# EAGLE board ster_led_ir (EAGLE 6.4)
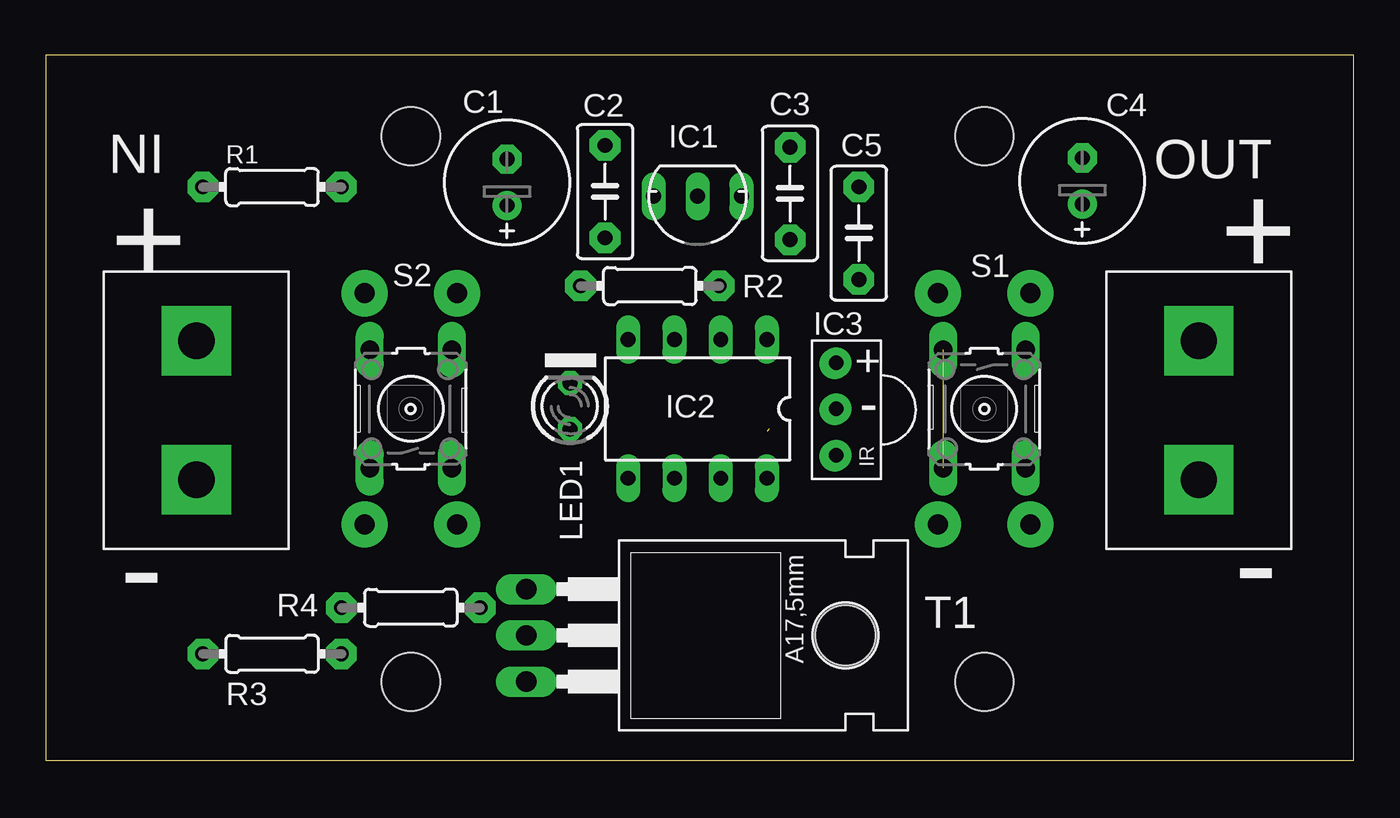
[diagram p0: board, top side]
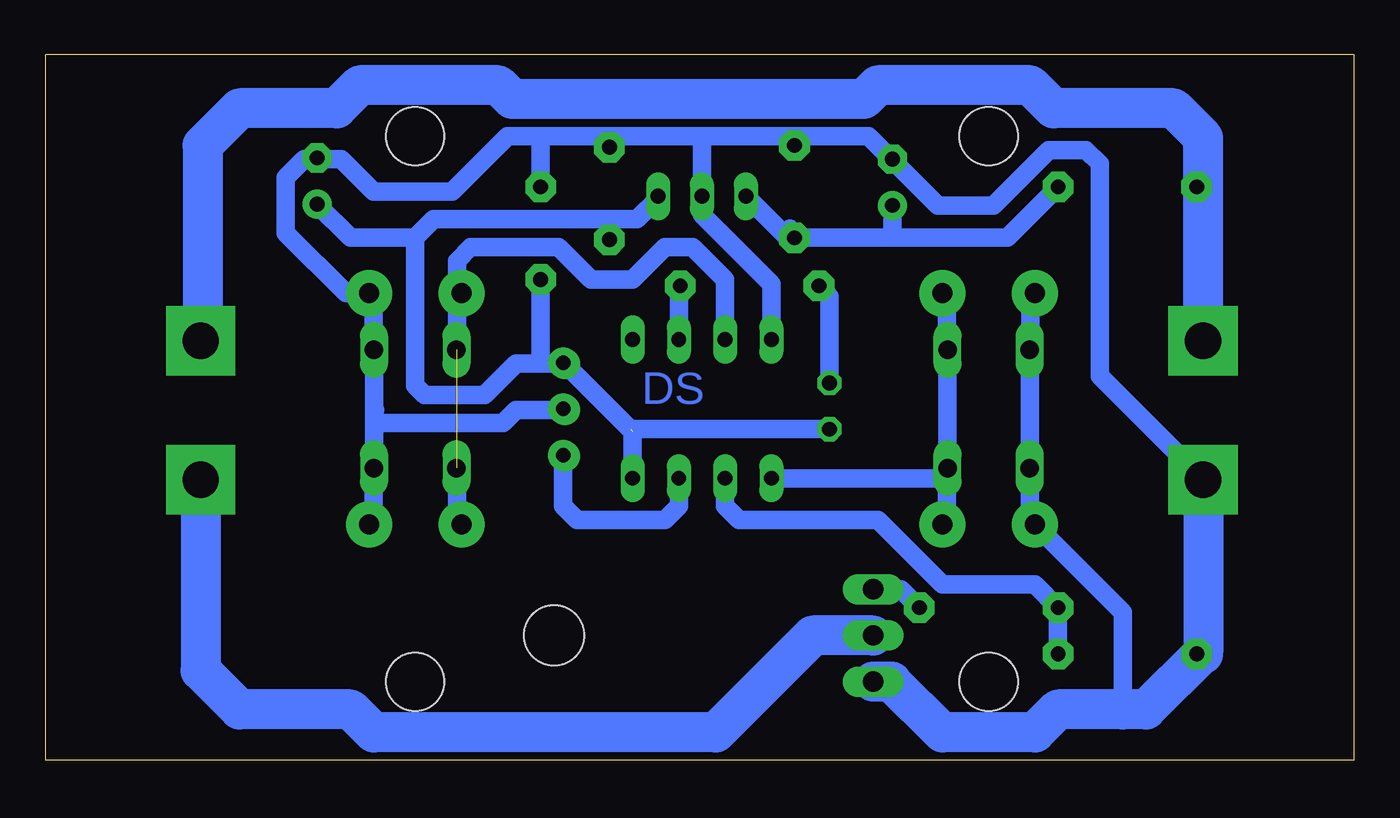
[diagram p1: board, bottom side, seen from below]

Size 71.87 x 38.76 mm. Coordinates in mm from the lower left corner, seen from the top.
Outline: 71.87,0 71.87,38.76 0,38.76 0,0 71.87,0
Copper layers (1*16): Top 0.035mm / dielectric 1.5mm / Bottom 0.035mm
Design rules "default": minimum track width 10mil, minimum drill 24mil, track to track 8mil, track to pad 8mil, pad to pad 8mil, via to via 8mil, smd to smd 8mil, copper to edge 40mil, drill to drill 8mil, minimum pad ring 10mil, minimum via ring 8mil, stop-mask expansion 4mil, vias tented up to drill 0mil, thermal gap 10mil
Holes 3.2 mm at 20.07,4.32 51.56,4.32 51.56,34.29 20.07,34.29

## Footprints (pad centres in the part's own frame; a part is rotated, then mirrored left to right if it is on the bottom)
E2,5-7 = drill 0.813 pad 1.6: + -1.27,0 | drill 0.813 pad 1.6 octagon: - 1.27,0
C050-030X075 = drill 0.813 pad 1.676 octagon: 1 -2.54,0; 2 2.54,0
78LXX = drill 0.813 long: GND 0,0; IN 2.413,0; OUT -2.413,0
DIL08 = drill 0.813 long: 1 -3.81,-3.81; 2 -1.27,-3.81; 3 1.27,-3.81; 4 3.81,-3.81; 5 3.81,3.81; 6 1.27,3.81; 7 -1.27,3.81; 8 -3.81,3.81
SFH5111 = drill 0.5 pad 1.676: GND 0,2.54; OUT 0,0; VCC 0,5.08
ARK2/750 = drill 2 pad 3.81 square: 1 -3.81,0; 2 3.81,0
LED3MM = drill 0.813 octagon: A -1.27,0; K 1.27,0
0204/7 = drill 0.813 pad 1.676 octagon: 1 -3.81,0; 2 3.81,0
B3F-10XX = drill 1.016 long: 1 -3.251,2.261; 2 3.251,2.261; 3 -3.251,-2.261; 4 3.251,-2.261
TO220 = drill 1.118 long: 1 -2.54,-6.35; 2 0,-6.35; 3 2.54,-6.35 | hole 3.302: 0,11.176

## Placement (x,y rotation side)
C1  100uF/35V  [E2,5-7]  25.35,31.75 90 top
C2  100nF  [C050-030X075]  30.73,31.24 90 top
C3  100nF  [C050-030X075]  40.89,31.14 90 top
C4  100uF/35V  [E2,5-7]  56.95,31.83 90 top
C5  100nF  [C050-030X075]  44.68,28.96 90 top
IC1  78L05  [78LXX]  35.81,30.99 180 top
IC2  ATTINY85  [DIL08]  35.81,19.3 180 top
IC3  [SFH5111]  43.36,16.71 0 top
IN  ARK2  [ARK2/750]  8.29,19.23 270 top
LED1  [LED3MM]  28.8,19.46 90 top
OUT  ARK2  [ARK2/750]  63.35,19.23 90 top
R1  100R  [0204/7]  12.45,31.5 0 top
R2  2,2k  [0204/7]  33.2,26.06 0 top
R3  2,2k  [0204/7]  12.45,5.84 180 top
R4  100R  [0204/7]  20.07,8.38 180 top
S1  [B3F-10XX]  51.56,19.3 270 top
S2  [B3F-10XX]  20.07,19.3 90 top
T1  IRL3803  [TO220]  32.77,6.86 270 top

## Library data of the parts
C1-C5 R1-R4 = rcl
IC1 = v-reg
IC2 = atmel; MPN: ATTINY13-20PU; OC_FARNELL: 9171550; OC_NEWARK: 96K6521
IC3 = sfh511x
IN OUT = dimmer
LED1 = led
S1 S2 = switch-omron; MPN: B3F-1000; OC_FARNELL: 176432; OC_NEWARK: 36M3542
T1 = transistor-fet

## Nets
+5V: C3.1 C4.+ C5.1 IC1.OUT IC2.8 IC3.VCC LED1.A
+12V: IN.1 OUT.2 R1.1
GND: C1.- C2.2 C3.2 C4.- C5.2 IC1.GND IC2.4 IC3.GND IN.2 R3.2 S1.1 S1.2 S2.1 S2.2 T1.3
IR: IC2.7 IC3.OUT
LED1: IC2.2 R2.2
N$1: R4.1 T1.1
N$2: C1.+ C2.1 IC1.IN R1.2
N$3: OUT.1 T1.2
N$13: LED1.K R2.1
PWM: IC2.6 R3.1 R4.2
S1: IC2.3 S1.3 S1.4
S2: IC2.5 S2.3 S2.4

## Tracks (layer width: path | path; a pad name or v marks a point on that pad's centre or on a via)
+5V  (1 unrouted)
  Bottom 1.016: C4.+ 56.95,30.53 55.12,28.7 51.56,28.7 | LED1.A 39.75,18.19 | 44.7,21.79 IC3.VCC 39.62,18.06 IC2.8 | 44.7,21.79 46.02,21.79 47.75,20.07 51.05,20.07 51.56,20.57 51.56,28.7 | C3.1 40.89,29.72 | 40.89,29.72 50.55,29.72 51.56,28.7 | IC1.OUT 38.23,30.86 39.37,29.72 40.89,29.72 | C5.1 44.68,21.82 44.7,21.79
+12V
  Bottom 1.016: R1.1 8.54,31.5 8.29,31.24
  Bottom 2.184: IN.1 8.29,31.24 8.29,34.2 9.91,35.81 16.51,35.81 17.78,37.08 26.16,37.08 26.92,36.32 46.23,36.32 46.99,37.08 54.61,37.08 55.88,35.81 61.21,35.81 63.25,33.78 63.25,23.14 OUT.2
GND  (via drill 1.1 pad 2.54)
  Bottom 1.016: R3.2 8.29,5.84 | 12.7,2.79 12.7,8.13 v17.53,12.95 17.8,13.23 S2.1 S2.2 | 25.4,33.02 22.86,30.48 19.81,30.48 16.76,33.53 14.73,33.53 13.97,32.77 13.97,21.1 IN.2 | C1.- 25.4,33.02 | 25.4,33.02 26.67,34.29 30.99,34.29 | 40.89,34.29 44.45,34.29 | 44.45,34.29 46.48,34.29 49.53,31.24 53.85,31.24 55.63,33.02 56.87,33.02 C4.- 57.02,33.02 57.66,33.02 58.67,32 58.67,28.96 55.37,25.65 54.1,25.65 53.85,25.4 53.85,22.58 S1.1 53.82,19.3 | 53.82,19.3 53.82,18.54 | 53.82,18.54 S1.2 | 53.77,19.25 53.82,19.3 | C3.2 40.89,34.29 | C5.2 44.68,34.27 44.45,34.29 | 30.99,34.29 35.81,34.29 | 35.81,34.29 40.89,34.29 | C2.2 30.73,34.04 30.99,34.29 | 35.81,34.29 IC1.GND 35.81,29.97 32,26.16 IC2.4 | IC3.GND 46.02,19.25 46.74,18.54 53.82,18.54
  Bottom 2.184: IN.2 8.29,5.94 | 8.29,5.84 8.29,5.94 | 8.29,5.94 11.43,2.79 12.7,2.79 16.26,2.79 17.53,1.52 22.61,1.52 25.4,4.32 T1.3
IR
  Bottom 1.016: IC2.7 37.08,13.97 37.85,13.21 42.67,13.21 43.43,13.97 43.43,16.64 IC3.OUT
LED1
  Bottom 1.016: IC2.2 37.08,25.98 R2.2
N$1
  Bottom 1.016: T1.1 24.89,9.4 R4.1
N$2
  Bottom 1.016: R1.2 19.05,28.7 25.4,28.7 | 25.4,28.7 31.11,28.7 31.3,28.89 | 31.3,28.89 IC1.IN | C2.1 30.99,29.21 31.3,28.89 | C1.+ 25.35,28.75 25.4,28.7
N$3
  Bottom 2.184: T1.2 29.72,6.86 35.05,1.52 53.85,1.52 55.12,2.79 61.21,2.79 63.35,4.93 OUT.1
N$4  (via drill 1.1 pad 2.54)
  Bottom 1.016: 17.78,22.61 17.78,25.4 v17.53,25.65
N$5  (via drill 1.1 pad 2.54)
  Bottom 1.016: 22.35,22.61 22.35,25.4 v22.61,25.65
N$6  (via drill 1.1 pad 2.54)
  Bottom 1.016: 22.35,16 22.35,13.21 v22.61,12.95
N$7  (via drill 1.1 pad 2.54)
  Bottom 1.016: 48.77,25.65 v49.02,25.65
N$8  (via drill 1.1 pad 2.54)
  other vias: 54.1,25.65
N$9  (via drill 1.1 pad 2.54)
  Bottom 1.016: 53.85,16 53.85,13.21 v54.1,12.95
N$10  (via drill 1.1 pad 2.54)
  Bottom 1.016: 49.28,16 49.28,13.21 v49.02,12.95
N$11  (via drill 0.8 pad 1.68)
  other vias: 43.43,21.84
N$12  (via drill 0.8 pad 1.68)
  other vias: 43.43,19.3
N$13
  Bottom 1.016: LED1.K 28.8,25.48 R2.1
N$14  (via drill 0.8 pad 1.68)
  other vias: 43.43,16.76
PWM
  Bottom 1.016: R3.1 R4.2 17.53,9.65 22.61,9.65 26.16,13.21 33.78,13.21 34.54,13.97 IC2.6
S1  (1 unrouted)
  Bottom 1.016: IC2.3 34.54,26.42 36.32,28.19 37.85,28.19 39.62,26.42 41.91,26.42 43.69,28.19 48.51,28.19 49.28,27.43 49.28,22.58 S1.3
S2
  Bottom 1.016: IC2.5 22.89,15.49 S2.3 S2.4

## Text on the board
Bottom: DS
tPlace: + | - | IR
tNames: + | + | IC3 | - | -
